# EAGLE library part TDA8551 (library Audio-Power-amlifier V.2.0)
1 W BTL audio amplifier with digital volume control
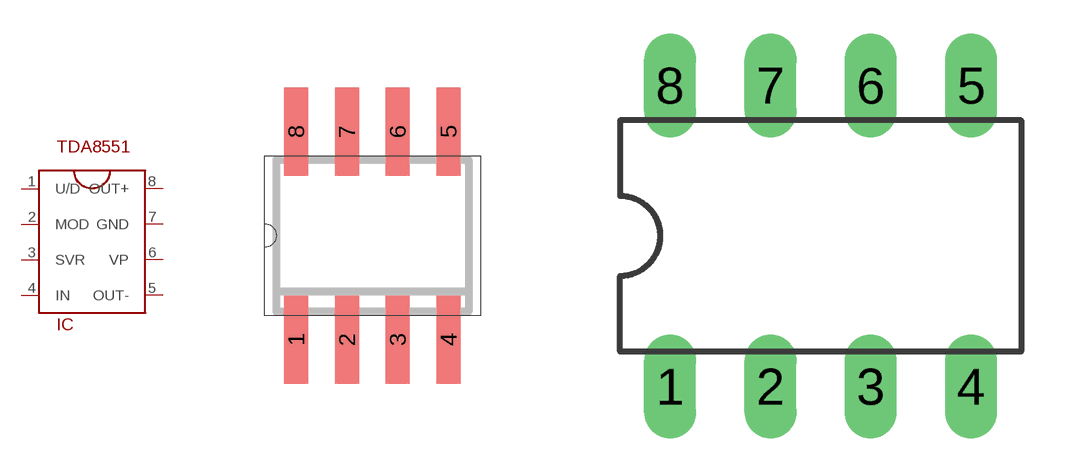
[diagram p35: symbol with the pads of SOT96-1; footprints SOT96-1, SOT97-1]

Designator prefix IC

## TDA8551  [SOT96-1]
1  U/D
2  MOD
3  SVR
4  IN  in
5  OUT-  out
6  VP  pwr
7  GND  pwr
8  OUT+  out

## TDA8551SOT97-1  [SOT97-1]
Pads as for SOT96-1

## Footprint SOT96-1 (pad centres in mm)
Small Outline Narrow Plastic Gull Wing 150-mil body, package type SN
smd 0.6 x 2.2: 1 -1.905,-2.6; 2 -0.635,-2.6; 3 0.635,-2.6; 4 1.905,-2.6; 5 1.905,2.6; 6 0.635,2.6; 7 -0.635,2.6; 8 -1.905,2.6

## Footprint SOT97-1 (pad centres in mm)
Dual In Line Package
drill 0.813 long: 1 -3.81,-3.81; 2 -1.27,-3.81; 3 1.27,-3.81; 4 3.81,-3.81; 5 3.81,3.81; 6 1.27,3.81; 7 -1.27,3.81; 8 -3.81,3.81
